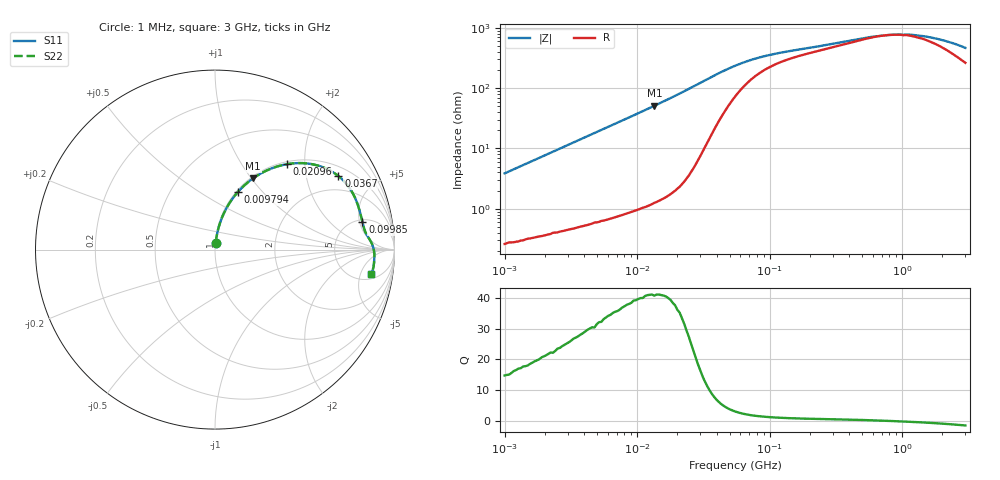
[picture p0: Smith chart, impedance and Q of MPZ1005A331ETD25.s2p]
! S-parameter Generated by TDK Corporation
! Copyright(C) 2018 TDK Corporation.
! All Rights Reserved.
! TDK P/N: MPZ1005A331ETD25 (Chip Bead)
! Property: |Z|=330¶ at 100MHz
! Size(LxWxT): 1x0.5x0.5mm, 0.039x0.02x0.02inches
! Model Type: s2p (Touchstone File Format Version 1.0)
! Frequency: DC=Yes Start=1MHz Stop=3000MHz 202points Log-sweep
! Model Generated on Aug. 6, 2018
! Port Assignments:
!  1 ---@@@--- 2
! Applicable Conditions:
!  Temperature = 25 degC
!  DC Bias Current = 0 A
!  Small Signal Operation
! Terms and conditions regarding TDK Simulation Models
! (1)This simulation model is being provided solely for informational purposes. Please refer to the specifications of the products in terms of detailed characteristics of such products.
! (2)In no event shall TDK Corporation of any of its subsidiaries be liable for any loss or damage arising, directly or indirectly,
!  From any information contained in this simulation model, including, but not limited to loss or damages arising from any inaccuracies, omissions or errors in connection with such information.
! (3)Any and all copyrights on this simulation model are owned by TDK Corporation.
!  Duplication or redistribution of this simulation model without prior written permission from TDK Corporation is prohibited.
! (4)This simulation model is subject to any modification or change without any prior notice.
! (5)Neither TDK Corporation nor any of its subsidiaries shall make any warranty, express or implied,
!  Including but not limited to the correctness, implied warranties of merchantability and fitness for a particular purpose with respect to this simulation models.
! (6)The use of this simulation model shall be deemed to have consented to the terms and conditions hereof.
# Hz S MA R 50
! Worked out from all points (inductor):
!   201 points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, 1 MHz to 3 GHz, reference 50 ohm
!   read as one part in series: L = 611 nH near 1.041 MHz
!   highest Q = 41 at 13.49 MHz (marker M1), where L = 602 nH
!   self-resonance near 810.1 MHz
!   S11 on the Smith chart (normalised r, x): 1 MHz: 1.01, +0.08; 9.794 MHz: 1.02, +0.74; 20.96 MHz: 1.05, +1.63; 36.7 MHz: 1.35, +3.08; 99.85 MHz: 5.47, +5.53; 3 GHz: 6.27, -7.71
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1000000  0.03846 83.9  0.9967 -2.2  0.9967 -2.2  0.03846 83.9
2055611  0.07794 82.9  0.9933 -4.5  0.9933 -4.5  0.07794 82.9
3900413  0.1451 79.7  0.9844 -8.3  0.9844 -8.3  0.1451 79.7
6563319  0.2381 74.6  0.9645 -13.8  0.9645 -13.8  0.2381 74.6
9794439  0.3429 68.5  0.9307 -20.0  0.9307 -20.0  0.3429 68.5
1.349163e7  0.4504 61.8  0.8819 -26.8  0.8819 -26.8  0.4504 61.8
1.461624e7  0.4802 59.9  0.8655 -28.7  0.8655 -28.7  0.4802 59.9
2.095589e7  0.6231 49.8  0.7646 -38.5  0.7646 -38.5  0.6231 49.8
2.459509e7  0.686 44.6  0.7029 -43.3  0.7029 -43.3  0.686 44.6
2.773354e7  0.7288 40.5  0.65 -46.7  0.65 -46.7  0.7288 40.5
3.670325e7  0.8003 30.8  0.5156 -52.7  0.5156 -52.7  0.8003 30.8
4.483659e7  0.8239 24.7  0.4267 -53.9  0.4267 -53.9  0.8239 24.7
5.477226e7  0.8324 19.7  0.3543 -52.4  0.3543 -52.4  0.8324 19.7
7.248696e7  0.8345 14.4  0.2831 -47.3  0.2831 -47.3  0.8345 14.4
9.984923e7  0.8356 10.5  0.2349 -40.5  0.2349 -40.5  0.8356 10.5
2.136344e8  0.8483 5.7  0.1773 -28.4  0.1773 -28.4  0.8483 5.7
5.81181e8  0.8785 1.6  0.1242 -11.1  0.1242 -11.1  0.8785 1.6
8.005644e8  0.8843 0.1  0.1157 -0.4  0.1157 -0.4  0.8843 0.1
1.10276e9  0.8885 -1.5  0.1143 12.0  0.1143 12.0  0.8885 -1.5
1.519029e9  0.8894 -3.4  0.1241 25.3  0.1241 25.3  0.8894 -3.4
2.092429e9  0.8888 -5.7  0.1451 37.2  0.1451 37.2  0.8888 -5.7
3e9  0.8812 -9.0  0.1888 46.7  0.1888 46.7  0.8812 -9.0
